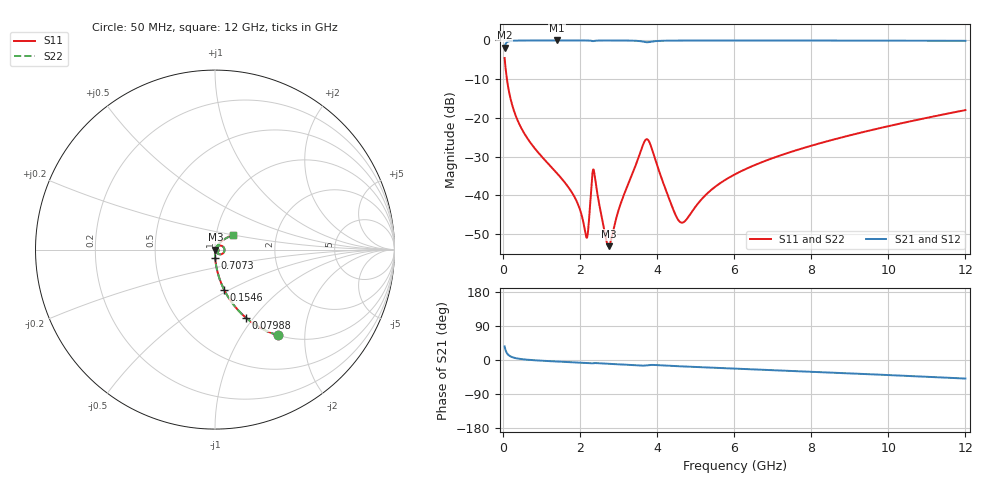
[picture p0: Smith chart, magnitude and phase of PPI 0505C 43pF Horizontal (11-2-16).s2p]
# MHz S MA R 50
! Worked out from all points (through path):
!   1601 points, 50 MHz to 12 GHz, reference 50 ohm
!   highest |S21| = -0.01 dB at 1.409 GHz (marker M1); lowest = -1.9 dB at 50 MHz (marker M2)
!   group delay of S21, straight-line fit = 12.1 ps
!   lowest |S11| = -53.1 dB at 2.746 GHz (marker M3), VSWR 1.00, Z = 50.2 - j0.041 ohm
!   |S11| at or under -10 dB: 110.2 MHz to end of sweep
!   |S22| runs from -53.1 to -4.5 dB; largest |S21 - S12| = 0
!   S11 on the Smith chart (normalised r, x): 50 MHz: 1.00, -1.47; 79.88 MHz: 1.00, -0.92; 154.6 MHz: 1.00, -0.47; 707.2 MHz: 1.00, -0.10; 12 GHz: 1.20, +0.19
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50  0.5926 -53.8  0.8053 36.2  0.8053 36.2  0.5926 -53.8
79.875  0.4181 -65.5  0.9081 24.4  0.9081 24.4  0.4181 -65.5
154.5625  0.2309 -77.1  0.9726 12.8  0.9726 12.8  0.2309 -77.1
363.6875  0.09905 -85.3  0.9945 4.4  0.9945 4.4  0.09905 -85.3
707.25  0.04878 -88.9  0.998 0.2  0.998 0.2  0.04878 -88.9
1409.312  0.01926 -91.0  0.9987 -4.0  0.9987 -4.0  0.01926 -91.0
1820.094  0.0104 -89.1  0.9986 -6.0  0.9986 -6.0  0.0104 -89.1
2044.156  0.005644 -80.5  0.9982 -7.1  0.9982 -7.1  0.005644 -80.5
2186.062  0.002848 -24.0  0.9971 -7.9  0.9971 -7.9  0.002848 -24.0
2320.5  0.01758 5.1  0.9828 -8.7  0.9828 -8.7  0.01758 5.1
2372.781  0.01993 -44.8  0.9838 -7.9  0.9838 -7.9  0.01993 -44.8
2656.594  0.003113 -52.8  0.9976 -9.5  0.9976 -9.5  0.003113 -52.8
2746.219  0.00221 -10.6  0.9976 -10.0  0.9976 -10.0  0.00221 -10.6
3687.281  0.05056 12.4  0.9545 -14.7  0.9545 -14.7  0.05056 12.4
3806.781  0.04839 -26.8  0.9527 -13.1  0.9527 -13.1  0.04839 -26.8
4038.312  0.0218 -60.2  0.9846 -13.7  0.9846 -13.7  0.0218 -60.2
4464.031  0.005872 -41.4  0.9944 -16.0  0.9944 -16.0  0.005872 -41.4
4643.281  0.004442 -5.3  0.9953 -16.8  0.9953 -16.8  0.004442 -5.3
6025  0.0187 58.5  0.9966 -22.7  0.9966 -22.7  0.0187 58.5
8019.156  0.04396 55.1  0.9956 -31.1  0.9956 -31.1  0.04396 55.1
10013.31  0.07842 47.8  0.993 -39.8  0.993 -39.8  0.07842 47.8
12000  0.126 39.3  0.9875 -49.0  0.9875 -49.0  0.126 39.3
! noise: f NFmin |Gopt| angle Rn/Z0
50  0.0003721  0.8591  0.6714  0.0005651
1372  0.003787  0.6601  5.101  0.002125
2701  0.007813  0.6741  9.826  0.004587
4031  0.02493  0.834  14.62  0.0312
5360  0.01301  0.6277  19.26  0.006374
6682  0.01387  0.5813  23.74  0.005793
8012  0.01548  0.5614  28.11  0.006
9341  0.01731  0.5517  32.35  0.006408
1.067e+04  0.01927  0.5482  36.44  0.006923
1.2e+04  0.02136  0.5492  40.38  0.007528
